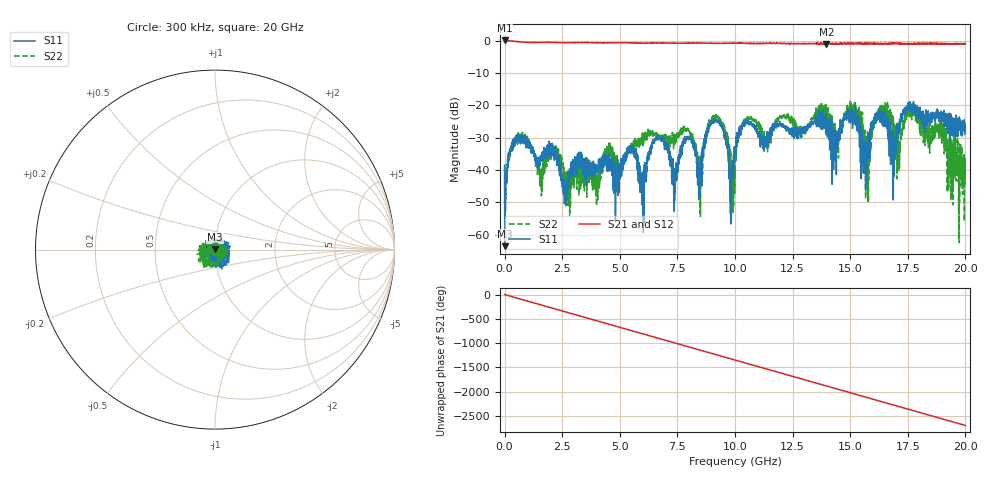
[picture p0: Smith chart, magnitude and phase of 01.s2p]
!Keysight Technologies,N5232A,MY52221221,A.10.65.11
!Date: Thursday, August 21, 2025 19:48:00
!Correction: S11(Full 2 Port(1,4))
!S41(Full 2 Port(1,4))
!S14(Full 2 Port(1,4))
!S44(Full 2 Port(1,4))
!S2P File: Measurements: S11, S41, S14, S44:
# Hz S  RI  R 50
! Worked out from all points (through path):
!   4001 points, 300 kHz to 20 GHz, reference 50 ohm
!   highest |S21| = 0.03 dB at 300 kHz (marker M1); lowest = -1.2 dB at 13.97 GHz (marker M2)
!   group delay of S21, straight-line fit = 374 ps
!   lowest |S11| = -63.6 dB at 5.3 MHz (marker M3), VSWR 1.00, Z = 50 + j0.0633 ohm
!   |S11| at or under -10 dB: start of sweep to end of sweep
!   |S22| runs from -62.6 to -18.7 dB; largest |S21 - S12| = 0.051
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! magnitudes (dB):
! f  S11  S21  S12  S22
! 300 kHz  -38.5  0.0  0.0  -38.9
! 5.3 MHz  -63.6  0.0  0.0  -54.2
! 680.3 MHz  -30.2  -0.4  -0.4  -29.6
! 2.625 GHz  -46.9  -0.6  -0.6  -40.9
! 3.335 GHz  -35.0  -0.6  -0.6  -40.0
! 5.49 GHz  -33.1  -0.7  -0.7  -31.8
! 5.97 GHz  -42.1  -0.8  -0.8  -30.1
! 6.67 GHz  -30.1  -0.7  -0.8  -29.7
! 7.955 GHz  -29.8  -0.8  -0.8  -27.5
! 8.48 GHz  -39.5  -0.7  -0.7  -43.6
! 9.245 GHz  -25.2  -0.9  -0.9  -24.1
! 9.83 GHz  -49.7  -0.8  -0.8  -36.9
! 10 GHz  -32.8  -0.8  -0.8  -40.2
! 10.5 GHz  -25.4  -0.9  -0.8  -24.5
! 13.34 GHz  -25.7  -1.0  -0.9  -24.6
! 13.97 GHz  -27.8  -1.2  -0.8  -24.1
! 15.2 GHz  -25.4  -0.9  -1.0  -21.6
! 15.77 GHz  -28.6  -1.0  -0.8  -49.7
! 16.67 GHz  -31.5  -1.0  -0.8  -23.5
! 17.06 GHz  -25.6  -0.9  -0.9  -39.4
! 17.72 GHz  -20.3  -1.0  -0.9  -21.1
! 20 GHz  -27.4  -1.0  -0.9  -36.5
